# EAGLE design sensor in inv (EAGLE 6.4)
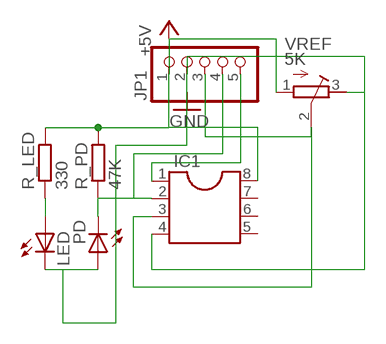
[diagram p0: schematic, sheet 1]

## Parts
IC1  DIL8S  [SOCKET-08]
JP1  PINHD-1X5  [1X05]
LED  LED3MM  [LED3MM]
PD  LED5MM  [LED5MM]
R_LED  330  R-EU_0204/7  [0204/7]
R_PD  47K  R-EU_0204/7  [0204/7]
VREF  5K  R-TRIMM64W  [RTRIM64W]

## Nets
+5V: IC1.8 JP1.1 R_LED.2 R_PD.2 VREF.1(A)
GND: IC1.4 JP1.2 LED.K(C) PD.A VREF.3(E)
N$1: LED.A R_LED.1
N$2: IC1.2 JP1.4 PD.K(C) R_PD.1
N$3: IC1.1 JP1.5
N$5: IC1.3 JP1.3 VREF.2(S)
Unconnected: IC1.5 IC1.6 IC1.7

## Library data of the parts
IC1 = ic-package:DIL8: Dual In Line / Socket
JP1 = pinhead:PINHD-1X5: PIN HEADER
LED PD = led:LED: LED
R_LED R_PD = rcl:R-EU_: RESISTOR, European symbol
VREF = rcl:R-TRIMM: Trimm resistor

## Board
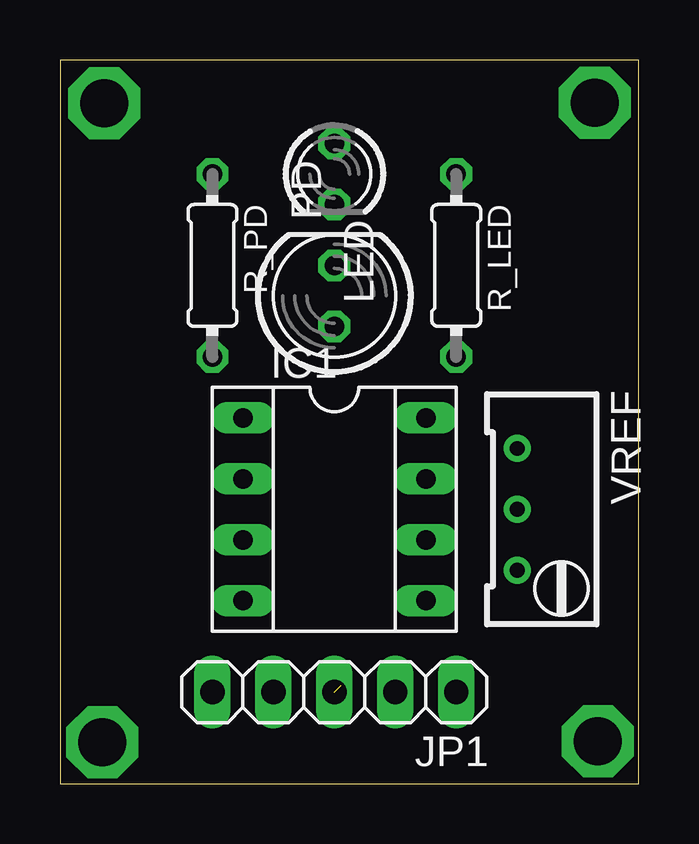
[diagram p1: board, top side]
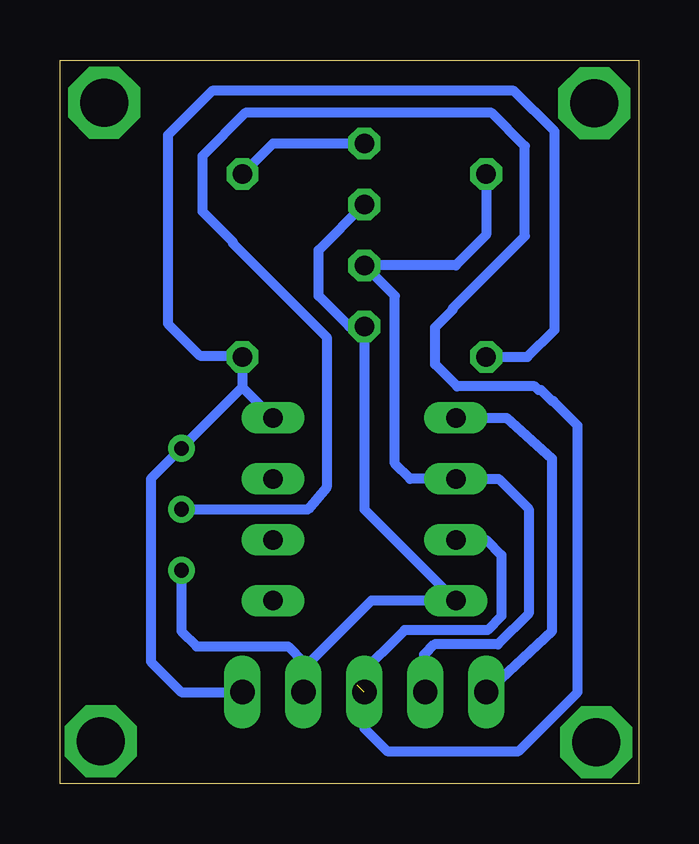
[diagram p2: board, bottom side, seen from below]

Size 24.11 x 30.15 mm. Coordinates in mm from the lower left corner, seen from the top.
Outline: 0,0 24.11,0 24.11,30.15 0,30.15 0,0
Copper layers (1*16): Top 0.035mm / dielectric 1.5mm / Bottom 0.035mm
Design rules "default": minimum track width 10mil, minimum drill 24mil, track to track 8mil, track to pad 8mil, pad to pad 8mil, via to via 8mil, smd to smd 8mil, copper to edge 40mil, drill to drill 8mil, minimum pad ring 10mil, minimum via ring 8mil, stop-mask expansion 4mil, vias tented up to drill 0mil, thermal gap 10mil

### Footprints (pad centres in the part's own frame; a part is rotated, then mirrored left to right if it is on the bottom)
SOCKET-08 = drill 0.813 long: 1 -3.81,-3.81; 2 -1.27,-3.81; 3 1.27,-3.81; 4 3.81,-3.81; 5 3.81,3.81; 6 1.27,3.81; 7 -1.27,3.81; 8 -3.81,3.81
1X05 = drill 1.016 long: 1 -5.08,0; 2 -2.54,0; 3 0,0; 4 2.54,0; 5 5.08,0
LED3MM = drill 0.813 octagon: A -1.27,0; K 1.27,0
LED5MM = drill 0.813 octagon: A -1.27,0; K 1.27,0
0204/7 = drill 0.813 octagon: 1 -3.81,0; 2 3.81,0
RTRIM64W = drill 0.61: 1 1.27,-2.54; 2 1.27,0; 3 1.27,2.54

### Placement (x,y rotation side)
IC1  11.43,11.43 270 top
JP1  11.43,3.81 180 top
LED  11.43,25.4 270 top
PD  11.43,20.32 90 top
R_LED  16.51,21.59 270 top
R_PD  6.35,21.59 270 top
VREF  20.32,11.43 180 top

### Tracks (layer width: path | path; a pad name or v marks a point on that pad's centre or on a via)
+5V
  Bottom 0.406: 16.51,16.51 R_LED.2 16.56,17.83 18.28,17.83 19.62,19.17 19.62,27.02 17.77,28.87 5.2,28.87 3.5,27.17 3.5,18.91 4.63,17.78 R_PD.2 | 16.51,16.51 IC1.8 | JP1.1 19.05,3.81 20.32,5.08 20.32,12.7 VREF.1 16.51,16.51
GND
  Bottom 0.406: LED.K 13.34,22.23 13.34,20.32 12.07,19.05 PD.A 11.43,11.43 IC1.4 11.14,7.62 13.97,4.79 | 13.97,4.79 13.97,5.08 14.61,5.72 18.42,5.72 19.05,6.35 VREF.3 | 13.97,4.79 JP1.2
N$1
  Bottom 0.406: LED.A 15.24,26.67 R_LED.1
N$2
  Bottom 0.406: R_PD.1 6.35,22.86 7.62,21.59 PD.K 10.16,20.32 10.16,13.34 9.53,12.7 IC1.2 5.84,12.7 4.58,11.45 4.58,7.08 5.86,5.8 8.52,5.8 8.94,5.37 8.94,3.86 JP1.4
N$3
  Bottom 0.406: IC1.1 5.51,15.24 3.61,13.54 3.61,6.35 JP1.5
N$4  (via drill 2)
  other vias: 1.84,28.34
N$5  (1 unrouted)
  Bottom 0.406: IC1.3 6.35,10.16 5.72,9.53 5.72,6.98 6.29,6.4 9.76,6.4 11.72,4.43 11.72,4.1 | JP1.3 11.43,2.3 10.48,1.35 5,1.35 2.54,3.81 2.54,14.92 3.55,15.93 3.61,15.93 4.07,16.39 4.17,16.39 4.32,16.55 7.56,16.55 8.48,17.47 8.48,19.01 7.76,19.73 7.76,19.78 4.73,22.81 4.73,26.56 6.12,27.94 16.39,27.94 18.18,26.15 18.18,23.84 16.9,22.55 16.9,22.5 13,18.6 13,12.34 13.79,11.41 18.94,11.41 VREF.2
N$6  (via drill 2)
  other vias: 22.28,28.38
N$7  (via drill 2)
  other vias: 22.41,1.76
N$8  (via drill 2)
  other vias: 1.77,1.73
